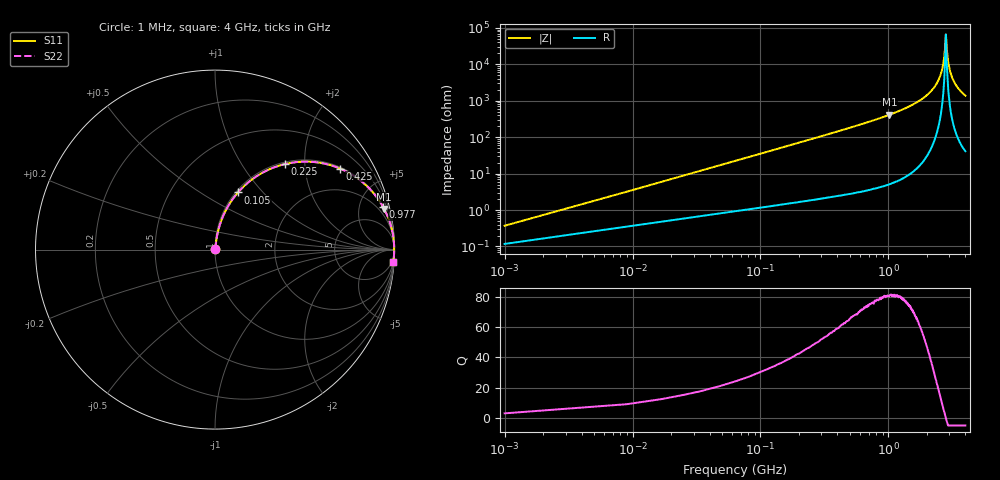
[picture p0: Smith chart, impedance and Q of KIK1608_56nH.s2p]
!version-2
!date-01.2022
!Series
# MHz S RI R 50
!Freq ReS11 ImS11 ReS21 ImS21 ReS12 ImS12 ReS22 ImS22
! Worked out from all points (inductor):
!   501 points, 1 MHz to 4 GHz, reference 50 ohm
!   read as one part in series: L = 56 nH near 17 MHz
!   highest Q = 80.9 at 1.02 GHz (marker M1), where L = 64.9 nH
!   self-resonance near 2.81 GHz
!   S11 on the Smith chart (normalised r, x): 1 MHz: 1.00, +0.01; 105 MHz: 1.02, +0.74; 225 MHz: 1.04, +1.59; 425 MHz: 1.05, +3.06; 977 MHz: 1.10, +7.82; 4 GHz: 2, -28
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1  0.00117 0.00351  0.9988 -0.00351  0.9988 -0.00351  0.00117 0.00351
25  0.0133 0.0863  0.9867 -0.0863  0.9867 -0.0863  0.0133 0.0863
33  0.0197 0.1131  0.9803 -0.1131  0.9803 -0.1131  0.0197 0.1131
65  0.0577 0.2136  0.9423 -0.2136  0.9423 -0.2136  0.0577 0.2136
105  0.1283 0.3187  0.8717 -0.3187  0.8717 -0.3187  0.1283 0.3187
225  0.3908 0.477  0.6092 -0.477  0.6092 -0.477  0.3908 0.477
425  0.6978 0.4511  0.3022 -0.4511  0.3022 -0.4511  0.6978 0.4511
673  0.8598 0.3405  0.1402 -0.3405  0.1402 -0.3405  0.8598 0.3405
977  0.9359 0.2387  0.064 -0.2387  0.064 -0.2387  0.9359 0.2387
1020  0.9428 0.2261  0.0572 -0.2261  0.0572 -0.2261  0.9428 0.2261
1335  0.9717 0.1597  0.0284 -0.1597  0.0284 -0.1597  0.9717 0.1597
2010  0.9937 0.069  0.00628 -0.069  0.00628 -0.069  0.9937 0.069
2450  0.9978 0.0282  0.00224 -0.0282  0.00224 -0.0282  0.9978 0.0282
2570  0.9982 0.0186  0.0018 -0.0186  0.0018 -0.0186  0.9982 0.0186
2670  0.9984 0.0106  0.00158 -0.0106  0.00158 -0.0106  0.9984 0.0106
2730  0.9985 0.00637  0.00153 -0.00637  0.00153 -0.00637  0.9985 0.00637
2815  0.9985 -1.29e-05  0.00151 1.29e-05  0.00151 1.29e-05  0.9985 -1.29e-05
2900  0.9984 -0.0062  0.00158 0.0062  0.00158 0.0062  0.9984 -0.0062
2980  0.9983 -0.0117  0.0017 0.0117  0.0017 0.0117  0.9983 -0.0117
3140  0.9979 -0.0222  0.00213 0.0222  0.00213 0.0222  0.9979 -0.0222
3335  0.9971 -0.0342  0.0029 0.0342  0.0029 0.0342  0.9971 -0.0342
4000  0.9927 -0.0715  0.0073 0.0715  0.0073 0.0715  0.9927 -0.0715
